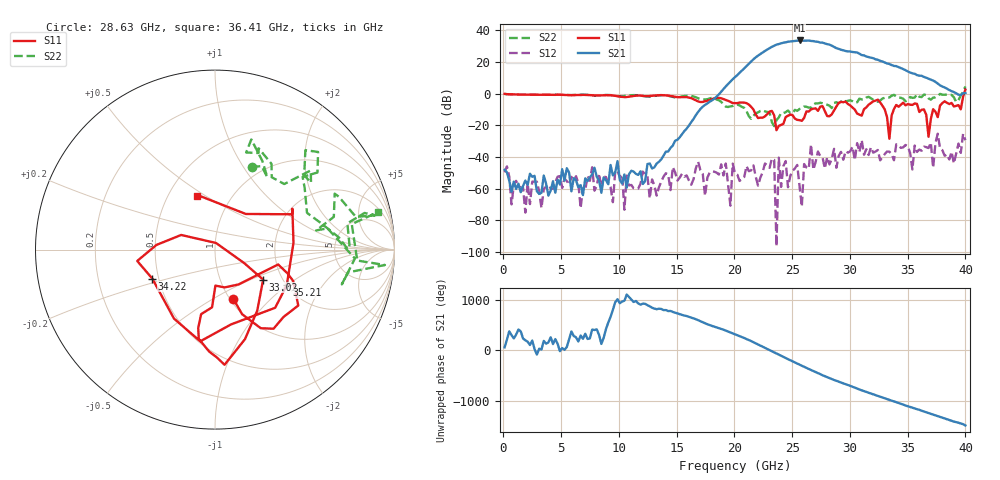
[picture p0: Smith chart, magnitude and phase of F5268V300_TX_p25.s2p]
!S2P File: Measurements: S11,S21,S12,S22
# MHz S  RI  R 50
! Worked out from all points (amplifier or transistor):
!   201 points, 100 MHz to 40 GHz, reference 50 ohm
!   highest |S21| = 33.6 dB at 25.64 GHz (marker M1)
!   |S21| within 3 dB of that: 23.54 GHz to 28.34 GHz (4.805 GHz wide, 18.5 % of centre)
!   unconditionally stable (mu >= 1): start of sweep to 26.56 GHz; 32.45 GHz to 37.78 GHz; 37.85 GHz to 39.68 GHz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
!   at 6.684 GHz: K = 42284.37, MAG = -42.0 dB, |S12| = -72.4 dB
!   at 20.05 GHz: K = 29.82, MAG = 12.6 dB, |S12| = -50.4 dB
!   at 40 GHz: K = 19.78, MSG = 14.9 dB, |S12| = -29.4 dB
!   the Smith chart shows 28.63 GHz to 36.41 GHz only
!   S11 on the Smith chart (normalised r, x): 28.63 GHz: 1.04, -0.63; 33.02 GHz: 1.60, -0.59; 34.22 GHz: 0.46, -0.17; 35.21 GHz: 2.01, -0.99; 36.41 GHz: 0.69, +0.46
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100  -0.9807 0.047  0.00216 0.00325  0.00322 -0.000393  -0.9772 0.0423
6883  -0.115 0.9062  -0.000415 -0.000462  0.00104 0.000168  -0.5436 0.7504
13467  0.8834 -0.0134  -0.00177 0.00679  -0.000773 0.00079  0.7662 0.43
20050  0.0248 -0.4989  2.412 -2.293  0.000342 0.00302  -0.0613 -0.4445
21646  -0.1138 -0.292  -11.43 4.093  0.00479 -0.00248  -0.1214 -0.1558
22444  -0.1628 0.0615  6.221 19.12  -0.00223 -0.00242  -0.2146 -0.2056
23242  -0.278 -0.0562  28.78 -8.716  0.00857 -0.00216  -0.1014 -0.0744
24040  0.087 -0.055  -12.41 -36.79  0.000368 -0.00106  -0.2269 0.0845
24838  0.1057 0.189  -42.2 13.97  -0.00225 0.00113  -0.2271 0.0868
25636  0.1226 0.077  12.86 46.01  0.000939 0.000754  -0.246 0.213
26235  0.273 -0.0159  46.3 8.546  -0.00218 0.00409  -0.2055 0.3233
26833  0.3184 -0.0994  27.51 -36.27  -0.00396 0.000197  -0.1146 0.4283
27831  0.2565 -0.1084  -34.63 -16.57  -0.00045 0.00429  0.0145 0.47
28629  0.103 -0.2761  -19.37 22.75  0.0142 0.0111  0.2035 0.4621
30025  0.4033 -0.1319  20.74 5.441  0.0137 0.00615  0.2431 0.5647
31222  -0.0164 -0.3216  -0.169 -16.13  0.000532 -0.0116  0.4971 0.4145
33018  0.2682 -0.1672  -5.553 7.807  0.00337 0.0118  0.739 0.00298
33417  0.00567 0.0369  -0.7977 8.604  0.000641 -0.0145  0.7375 0.1462
34215  -0.3496 -0.1611  5.758 3.753  -0.0211 0.00998  0.6896 0.295
35212  0.3999 -0.1981  3.343 -3.196  0.00852 -0.0104  0.7794 -0.0496
36409  -0.1023 0.2987  -2.362 -2.4  -0.00742 0.0198  0.9078 0.2085
40000  0.2721 -1.308  0.6499 -0.8179  -0.0233 -0.0245  1.418 -0.9065
